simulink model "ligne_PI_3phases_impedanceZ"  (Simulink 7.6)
settings: Solver=ode23t  StartTime=0.0  StopTime=2.5e-3  RelTol=1e-3
InitFcn:
  | clc
  | close all
  | clear all
  | delete *.mat
StopFcn:
  | close all
  | load IsA_VsA.mat
  | plotyy(x(1,:),x(2,:),x(1,:),x(3,:))
  | grid
  | title('Courant et tension Phase A')
  | xlabel('temps')
libraries: powerlib x8

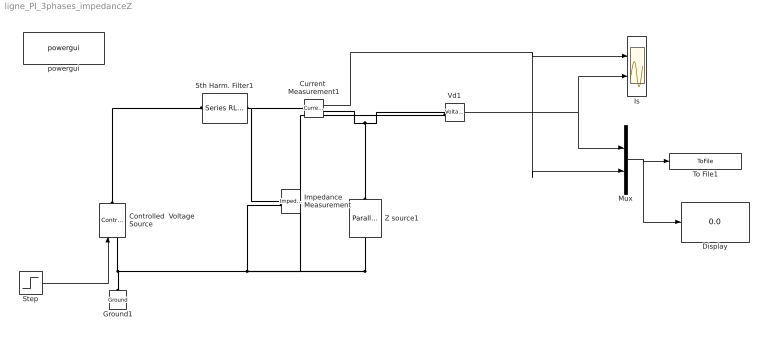
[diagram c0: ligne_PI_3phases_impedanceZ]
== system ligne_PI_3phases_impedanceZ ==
  5th Harm. Filter1 : powerlib/Elements/Series RLC Branch  DialogController=POWERSYS.PowerSysDialog  PhysicalDomain=powersysdomain  SubClassName=unknown  LeftPortType=p1  RightPortType=p1  LConnTagsString=__new0  RConnTagsString=__new0  BranchType=RLC  Resistance=1.27  Inductance=107.42e-03  SetiL0=off  InitialCurrent=0  Capacitance=2.62e-06  Setx0=off  InitialVoltage=0  Measurements=None
  Controlled  Voltage Source : powerlib/Electrical Sources/Controlled Voltage Source  DialogController=POWERSYS.PowerSysDialog  SystemSampleTime=-1  Initialize=on  Source_Type=AC  Amplitude=0  Phase=0  Frequency=0  Measurements=None
  Current  Measurement1 : powerlib/Measurements/Current Measurement  DialogController=POWERSYS.PowerSysDialog  SystemSampleTime=-1  PhasorSimulation=off  OutputType=Complex  PSBequivalent=0
  Display : Display
  Ground1 : powerlib/Elements/Ground  DialogController=POWERSYS.PowerSysDialog  PhysicalDomain=powersysdomain  SubClassName=unknown  LeftPortType=p1  RightPortType=p1  LConnTagsString=a
  Impedance  Measurement : powerlib/Measurements/Impedance Measurement  DialogController=POWERSYS.PowerSysDialog  PhysicalDomain=powersysdomain  SubClassName=unknown  LeftPortType=p1  RightPortType=p1  LConnTagsString=+|-  Factor=1
  Is : Scope  NumInputPorts=2
  Mux : Mux  Inputs=2
  Step : Step  Time=0  After=12  SampleTime=0
  To File1 : ToFile  Filename=IsA_VsA  MatrixName=x
  Vd1 : powerlib/Measurements/Voltage Measurement  Tag=PoWeRsYsTeMmEaSuReMeNt  DialogController=POWERSYS.PowerSysDialog  SystemSampleTime=-1  PhasorSimulation=off  OutputType=Magnitude  PSBequivalent=0
  Z source1 : powerlib/Elements/Parallel RLC Branch  DialogController=POWERSYS.PowerSysDialog  PhysicalDomain=powersysdomain  SubClassName=unknown  LeftPortType=p1  RightPortType=p1  LConnTagsString=a  RConnTagsString=__new0  BranchType=RLC  Resistance=37.7  Inductance=10e-03  SetiL0=off  InitialCurrent=0  Capacitance=0  Setx0=off  InitialVoltage=0  Measurements=None
  powergui : powerlib/powergui  Priority=1  SystemSampleTime=-1  SimulationMode=Continuous  SampleTime=1e-5  frequency=60  SPID=off  DisableSnubberDevices=off  DisableRonSwitches=off  DisableVfSwitches=off  SwTol=0  Interpol=off  frequencyindice=0  echomessages=off  HookPort=off  DisplayEquations=off  FunctionMessages=off  EnableUseOfTLC=off  x0status=blocks  RestoreLinks=warning  ResistiveCurrentMeasurement=off  Ylog=off  Xlog=on  ShowGrid=off  save=off  variable=ZData  ZoomFFT=off  StartTime=0.0  cycles=1  DisplayStyle=1  fundamental=60  FreqAxis=off  MaxFrequency=1000  frequencyindicesteady=1  display=off  methode=off
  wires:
  Mux/1 -> To File1/1, Display/1
  Step/1 -> Controlled  Voltage Source/1
  Current  Measurement1/1 -> Is/1, Mux/2
  Vd1/1 -> Is/2, Mux/1
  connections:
  Vd1/LConn2 -- Z source1/LConn1 -- Controlled  Voltage Source/LConn1 -- Ground1/LConn1 -- Impedance  Measurement/LConn2
  Controlled  Voltage Source/RConn1 -- 5th Harm. Filter1/RConn1
  Z source1/RConn1 -- Vd1/LConn1 -- Current  Measurement1/RConn1
  5th Harm. Filter1/LConn1 -- Current  Measurement1/LConn1 -- Impedance  Measurement/LConn1
